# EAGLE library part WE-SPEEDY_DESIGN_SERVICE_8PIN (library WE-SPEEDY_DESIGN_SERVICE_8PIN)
WE-Speedy Design Service, 8 Pin - Any application that fits package style - Switch Mode Power: Flyback, Forward, Push-Pull, Coupled Inductor -- Telecom Applications: xDSL, POTS Splitter Inductors
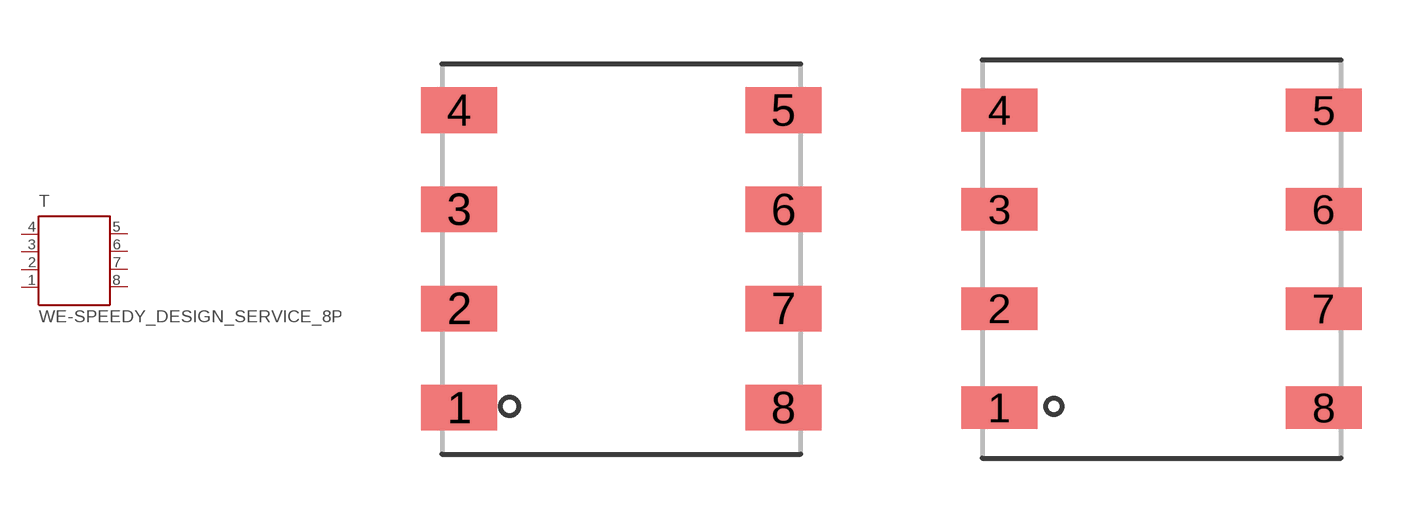
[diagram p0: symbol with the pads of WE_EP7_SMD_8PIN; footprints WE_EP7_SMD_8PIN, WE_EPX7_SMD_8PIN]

Designator prefix T

## WE-SPEEDY_DESIGN_SERVICE_8PIN_EP7_SMD  [WE_EP7_SMD_8PIN]
1  1  pas
2  2  pas
3  3  pas
4  4  pas
5  5  pas
6  6  pas
7  7  pas
8  8  pas

## WE-SPEEDY_DESIGN_SERVICE_8PIN_EPX7_SMD  [WE_EPX7_SMD_8PIN]
Pads as for WE_EP7_SMD_8PIN

## WE-SPEEDY_DESIGN_SERVICE_8PIN-750311342_EP10_SMD (MPN: 750311342; OC_FARNELL: 1895749; OC_NEWARK: 47T5827; PACKAGE: EP10-SMD; SUPPLIER: Würth Elektronik eiSos GmbH)  [WE_EP10_SMD_8PIN]
Pads as for WE_EP7_SMD_8PIN

## WE-SPEEDY_DESIGN_SERVICE_8PIN_EPX9_SMD  [WE_EPX9_SMD_8PIN]
Pads as for WE_EP7_SMD_8PIN

## WE-SPEEDY_DESIGN_SERVICE_8PIN_ER9.5_SMD  [WE_ER9.5_SMD_8PIN]
Pads as for WE_EP7_SMD_8PIN

## WE-SPEEDY_DESIGN_SERVICE_8PIN_EE13/5/6_THT  [WE_EE13/5/6_HORIZONTAL_8PIN]
1  4  pas
2  3  pas
3  2  pas
4  1  pas
5  8  pas
6  7  pas
7  6  pas
8  5  pas

## WE-SPEEDY_DESIGN_SERVICE_8PIN_EE13/7/5_THT  [WE_EE13/7/4_HORIZONTAL_8PIN]
Pads as for WE_EE13/5/6_HORIZONTAL_8PIN

## WE-SPEEDY_DESIGN_SERVICE_8PIN_EE16/8/5_THT  [WE_EE16/8/5_THT_HORIZONTAL_8PIN]
Pads as for WE_EE13/5/6_HORIZONTAL_8PIN

## WE-SPEEDY_DESIGN_SERVICE_8PIN_EE25/13/11_THT  [WE_EE25/13/11_THT_VERTICAL_8PIN]
Pads as for WE_EE13/5/6_HORIZONTAL_8PIN

## Footprint WE_EP7_SMD_8PIN (pad centres in mm)
Transformer, EP7 SMD 8 Pin
smd 1.91 x 1.143: 1 -4.065,-3.735; 2 -4.065,-1.245; 3 -4.065,1.245; 4 -4.065,3.735; 5 4.065,3.735; 6 4.065,1.245; 7 4.065,-1.245; 8 4.065,-3.735

## Footprint WE_EPX7_SMD_8PIN (pad centres in mm)
Transformer, EPX7 SMD 8 Pin
smd 1.91 x 1.07: 1 -4.065,-3.735; 2 -4.065,-1.245; 3 -4.065,1.245; 4 -4.065,3.735; 5 4.065,3.735; 6 4.065,1.245; 7 4.065,-1.245; 8 4.065,-3.735

## Footprint WE_EP10_SMD_8PIN (pad centres in mm)
Transformer, EP10 SMD 8 Pin
smd 2.08 x 1.07: 1 -6.78,-3.735; 2 -6.78,-1.245; 3 -6.78,1.245; 4 -6.78,3.735; 5 6.78,3.735; 6 6.78,1.245; 7 6.78,-1.245; 8 6.78,-3.735

## Footprint WE_EPX9_SMD_8PIN (pad centres in mm)
Transformer, EPX9 SMD 8 Pin
smd 2.44 x 0.97: 1 -4.13,-3; 2 -4.13,-1; 3 -4.13,1; 4 -4.13,3; 5 4.13,3; 6 4.13,1; 7 4.13,-1; 8 4.13,-3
